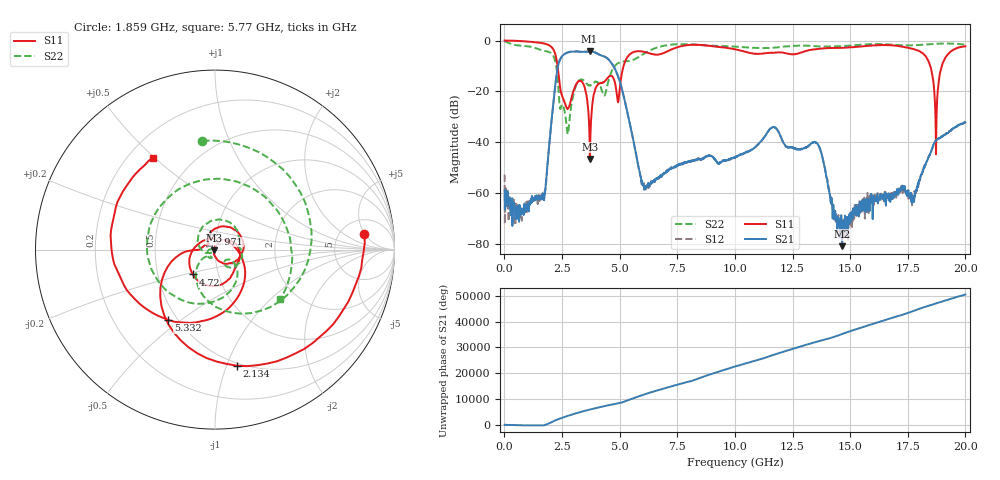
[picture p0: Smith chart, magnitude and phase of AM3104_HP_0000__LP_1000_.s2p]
!Created with skrf (http://scikit-rf.org).
# Hz S RI R 50.0
!freq ReS11 ImS11 ReS21 ImS21 ReS12 ImS12 ReS22 ImS22
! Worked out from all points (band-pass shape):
!   1601 points, 10 MHz to 20 GHz, reference 50 ohm
!   highest |S21| = -4.23 dB at 3.696 GHz (marker M1); lowest = -80.7 dB at 14.65 GHz (marker M2)
!   |S21| within 3 dB of the highest: 2.426 GHz to 4.5 GHz (2.074 GHz wide, 59.9 % of centre)
!   lowest |S11| = -46.5 dB at 3.708 GHz (marker M3), VSWR 1.01, Z = 49.6 - j0.285 ohm
!   |S11| at or under -10 dB: 2.307 GHz to 5.171 GHz (2.864 GHz wide, 76.6 % of centre); 18.48 GHz to 18.98 GHz (500.3 MHz wide, 2.67 % of centre)
!   |S22| runs from -36.7 to -0.2 dB; largest |S21 - S12| = 0.0051
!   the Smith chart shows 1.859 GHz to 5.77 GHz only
!   S11 on the Smith chart (normalised r, x): 1.859 GHz: 8.52, +4.78; 2.134 GHz: 0.48, -1.09; 2.971 GHz: 0.93, +0.17; 4.72 GHz: 0.75, -0.22; 5.332 GHz: 0.45, -0.45; 5.77 GHz: 0.30, +0.49
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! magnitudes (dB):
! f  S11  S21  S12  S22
! 10 MHz  0.0  -58.8  -52.6  -0.2
! 759.6 MHz  -0.2  -67.3  -70.7  -2.1
! 1.859 GHz  -1.6  -49.6  -50.0  -4.3
! 2.134 GHz  -3.6  -23.6  -23.6  -6.2
! 2.721 GHz  -26.7  -4.8  -4.8  -35.4
! 2.971 GHz  -20.6  -4.4  -4.4  -22.0
! 3.346 GHz  -16.0  -4.4  -4.4  -15.3
! 3.696 GHz  -38.8  -4.2  -4.2  -17.7
! 3.708 GHz  -46.5  -4.3  -4.2  -17.6
! 4.72 GHz  -14.6  -9.9  -9.9  -10.9
! 5.332 GHz  -6.6  -28.0  -27.9  -8.1
! 5.77 GHz  -4.2  -47.3  -47.5  -6.8
! 6.682 GHz  -5.5  -53.6  -54.0  -2.6
! 10.01 GHz  -3.4  -45.7  -46.0  -2.4
! 11.65 GHz  -4.8  -34.0  -33.9  -2.8
! 13.34 GHz  -3.6  -40.2  -40.2  -2.2
! 14.65 GHz  -2.9  -80.7  -73.6  -2.2
! 16.68 GHz  -1.8  -62.7  -61.8  -1.5
! 18.25 GHz  -5.8  -49.1  -49.1  -1.6
! 18.73 GHz  -44.6  -39.2  -39.2  -1.3
! 19.09 GHz  -7.5  -37.1  -37.0  -1.2
! 20 GHz  -2.3  -32.1  -32.0  -1.6
